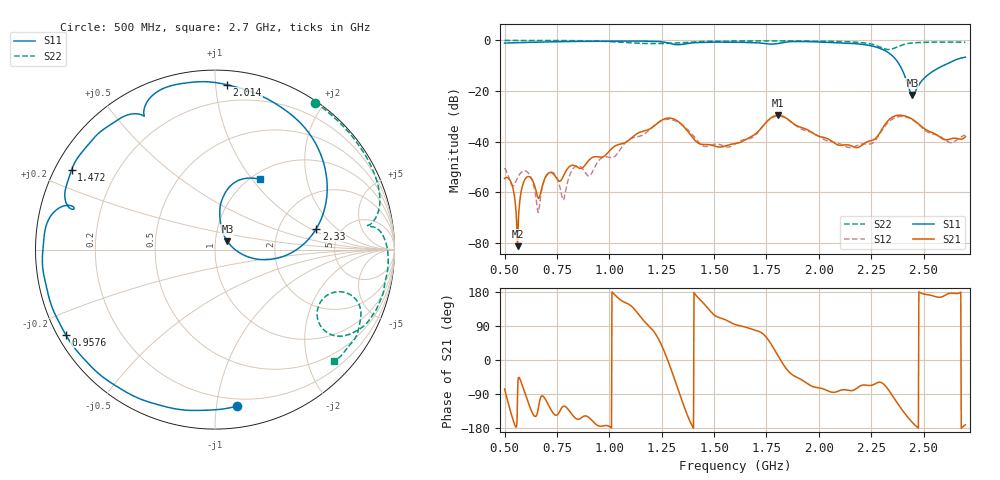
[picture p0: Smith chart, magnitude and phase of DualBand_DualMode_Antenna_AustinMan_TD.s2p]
! TOUCHSTONE file generated by CST MICROWAVE STUDIO
! Date and time: Mon May 18 00:08:47 2020
! Project name: DualBand_DualMode_Antenna_AustinMan_TD.cst
! Parameters = {FPL=20; FPW=20; L=50; ST=10; SW=30; W=55; WF=7; ext=10; gap=1; inset=20}
! Header version: 2015
! Port assignment regex: !\s*Touchstone port\s*([0-9]+)\s*=\s*CST MWS port\s*([0-9]+)\s*\(\"(.*)\"\)(\s*mode\s*([0-9]+))?.*
! Touchstone port assignment:
! Touchstone port 1 = CST MWS port 1 ("")
! Touchstone port 2 = CST MWS port 2 ("")
# GHz S MA R 50
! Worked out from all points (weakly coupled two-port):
!   1001 points, 500 MHz to 2.7 GHz, reference 50 ohm
!   highest |S21| = -29.61 dB at 1.807 GHz (marker M1); lowest = -81.4 dB at 561.6 MHz (marker M2)
!   lowest |S11| = -21.6 dB at 2.447 GHz (marker M3), VSWR 1.18, Z = 57.2 + j5.23 ohm
!   |S11| at or under -10 dB: 2.388 GHz to 2.595 GHz (207.4 MHz wide, 8.32 % of centre)
!   |S22| runs from -3.7 to -0.1 dB; largest |S21 - S12| = 0.0034
!   S11 on the Smith chart (normalised r, x): 500 MHz: 0.15, -1.14; 957.6 MHz: 0.02, -0.26; 1.472 GHz: 0.05, +0.26; 2.014 GHz: 0.09, +1.07; 2.33 GHz: 3.29, +1.16; 2.7 GHz: 1.09, +1.09
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0.5  0.8803 -82.2  0.001864 -76.5  0.003016 -157.1  0.9915 55.7
0.533  0.8897 -87.6  0.001485 -144.6  0.001403 94.7  0.9915 51.8
0.5616  0.8949 -92.1  8.551e-05 -99.2  0.001912 -26.4  0.9913 48.6
0.6056  0.9066 -98.9  0.00197 -101.4  0.002549 -128.3  0.9913 44.1
0.6606  0.9176 -107.5  0.0007602 -128.9  0.0003937 48.2  0.9908 38.9
0.7112  0.9284 -115.0  0.002399 -120.8  0.002386 -114.3  0.9896 34.6
0.7794  0.9379 -125.2  0.002023 -122.4  0.0007005 -147.3  0.9869 29.2
0.8234  0.946 -131.5  0.003391 -145.0  0.002772 -127.4  0.9835 25.9
0.8674  0.9494 -137.9  0.00296 -152.1  0.003044 -169.4  0.979 22.8
0.9576  0.9576 -150.4  0.004894 -174.9  0.004538 -161.0  0.9592 16.7
1.2348  0.9478 171.2  0.02384 55.4  0.02415 55.5  0.8621 8.9
1.4724  0.9144 150.9  0.008692 135.2  0.008115 141.2  0.9498 2.9
1.6  0.9173 135.5  0.009078 93.7  0.008901 101.9  0.966 -2.9
1.8068  0.8666 117.2  0.03309 9.9  0.03157 12.0  0.9642 -11.1
1.9674  0.9365 93.0  0.01506 -69.2  0.01498 -64.5  0.9627 -17.9
2.0136  0.9208 85.8  0.0123 -75.0  0.01166 -76.0  0.9595 -20.1
2.1874  0.8476 55.0  0.007623 -72.2  0.008497 -70.7  0.9091 -29.9
2.3304  0.5771 11.7  0.02575 -76.9  0.02364 -75.8  0.656 -27.8
2.3348  0.5608 10.0  0.02687 -80.3  0.02461 -79.0  0.6563 -26.4
2.447  0.08289 33.2  0.02751 -165.1  0.02679 -162.7  0.8868 -23.5
2.623  0.3599 76.9  0.01103 175.9  0.009633 172.2  0.9183 -36.9
2.7  0.4643 57.6  0.01246 -170.9  0.01354 -175.1  0.907 -43.3
